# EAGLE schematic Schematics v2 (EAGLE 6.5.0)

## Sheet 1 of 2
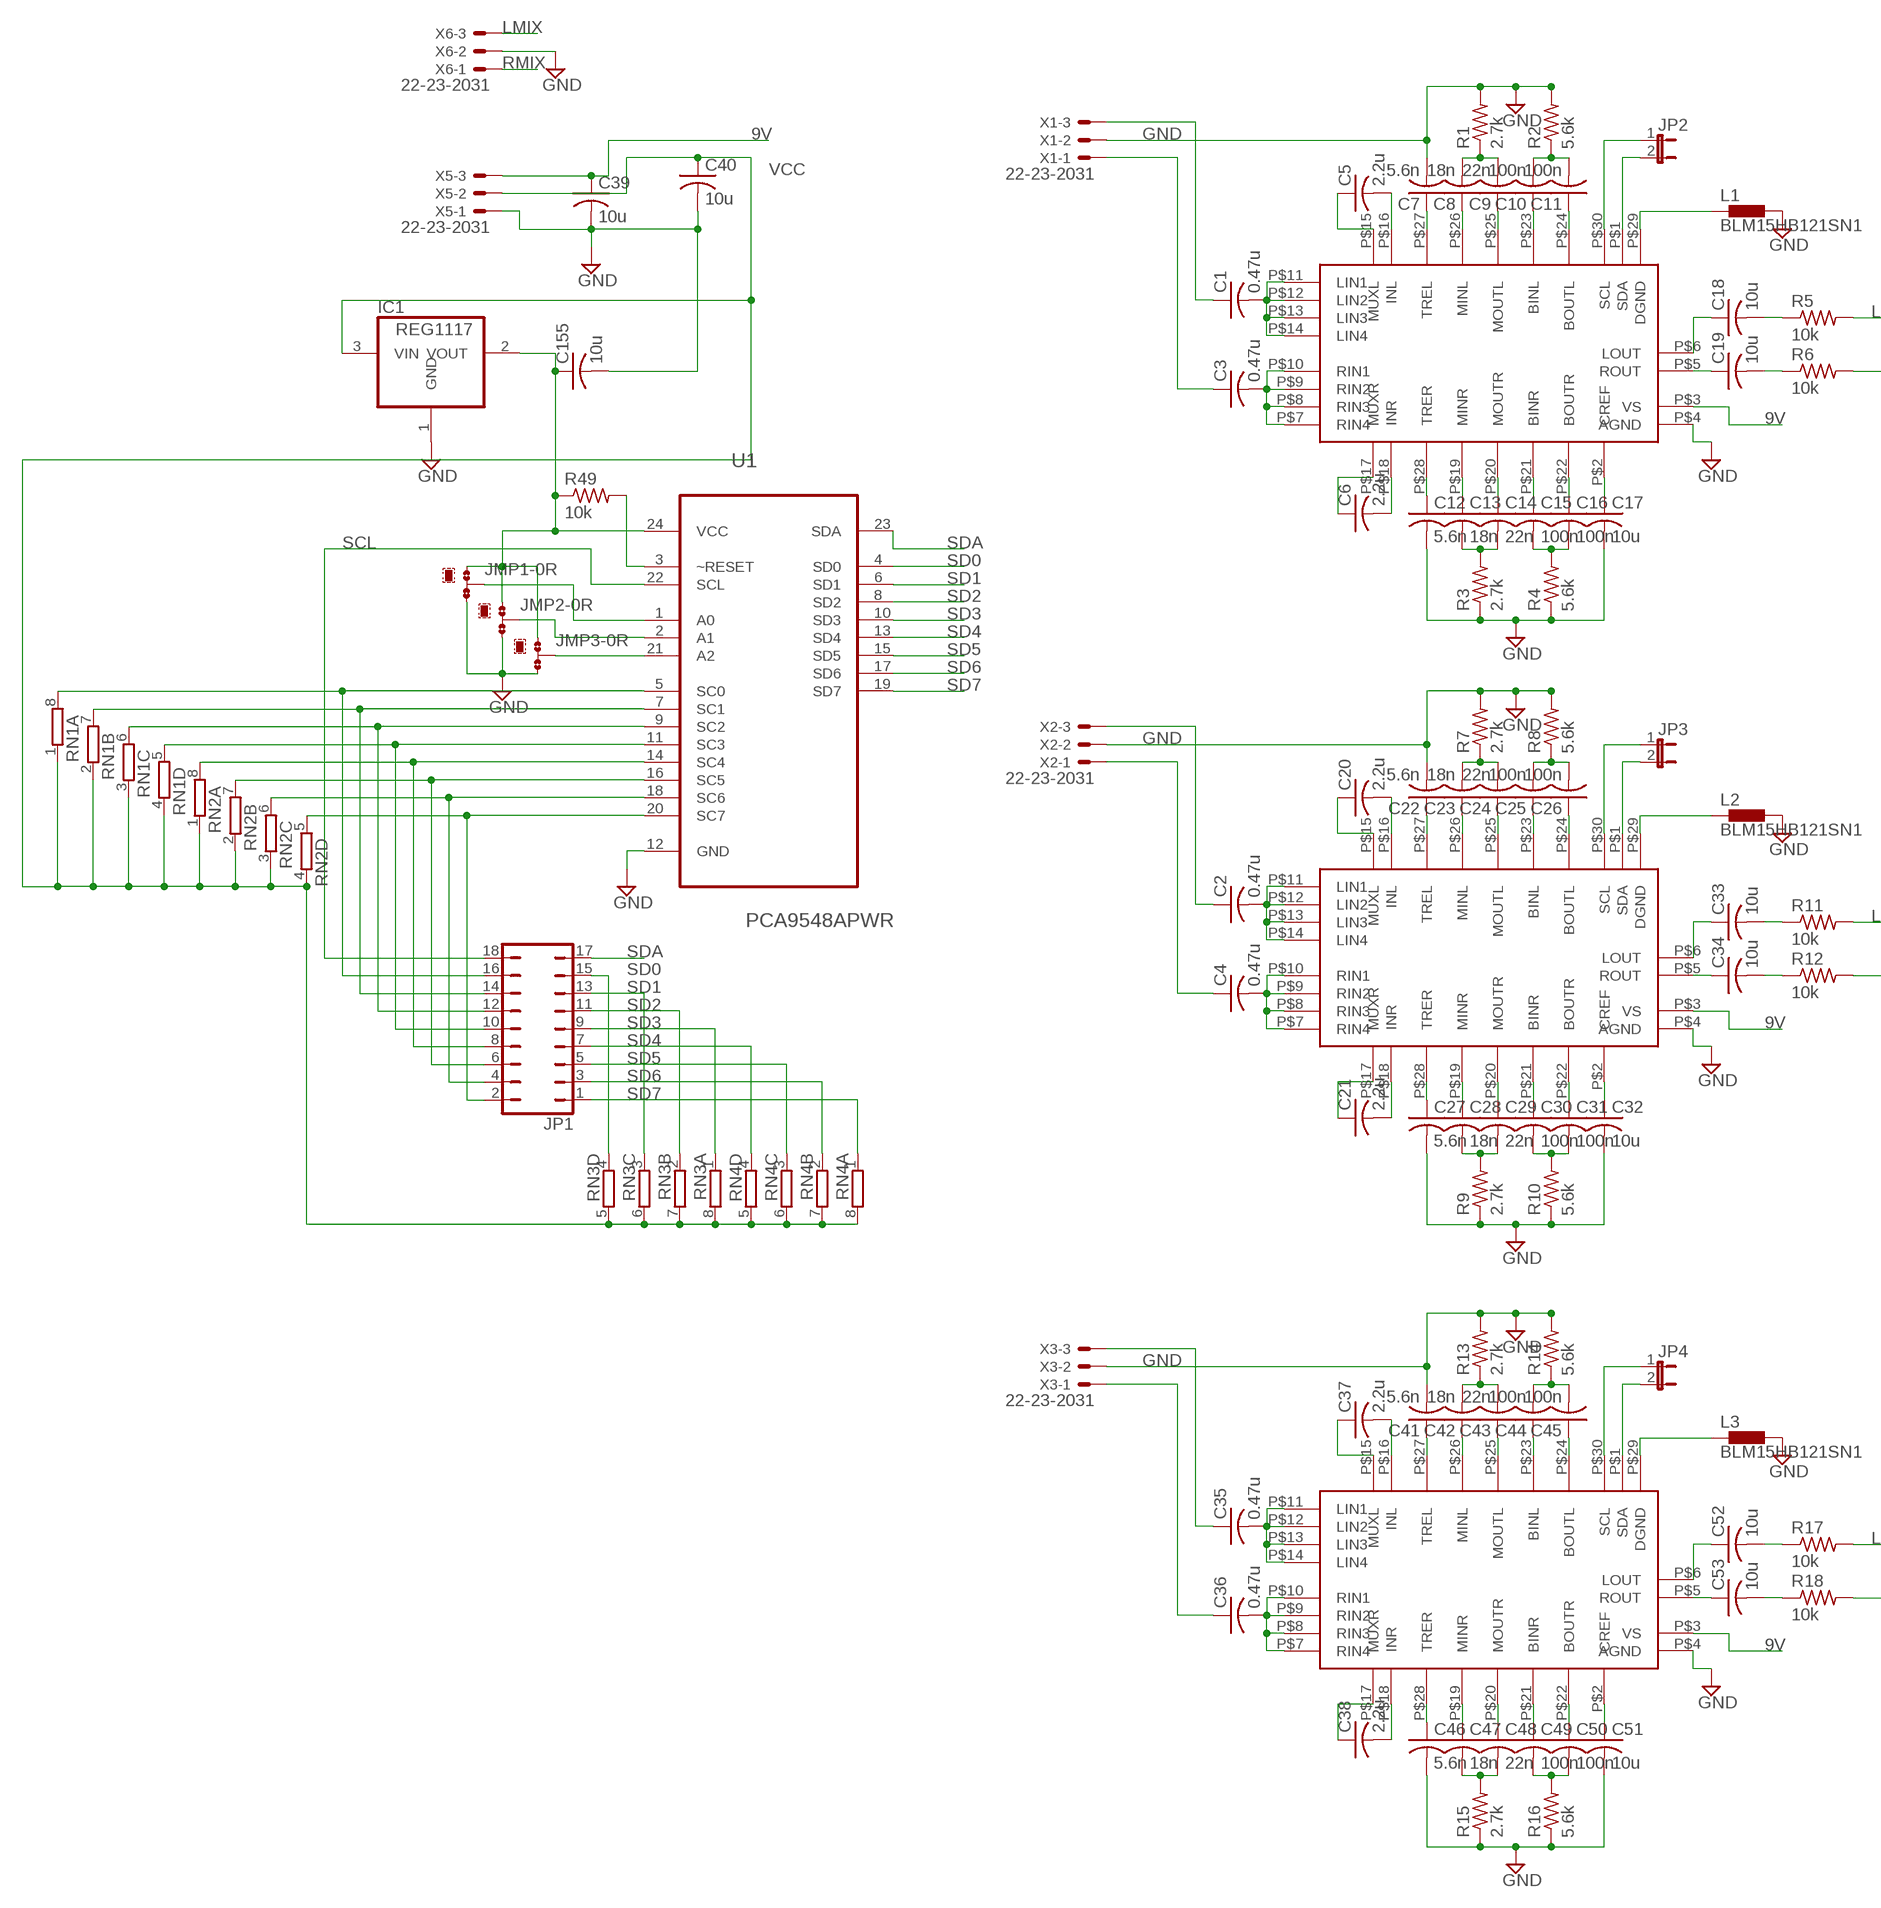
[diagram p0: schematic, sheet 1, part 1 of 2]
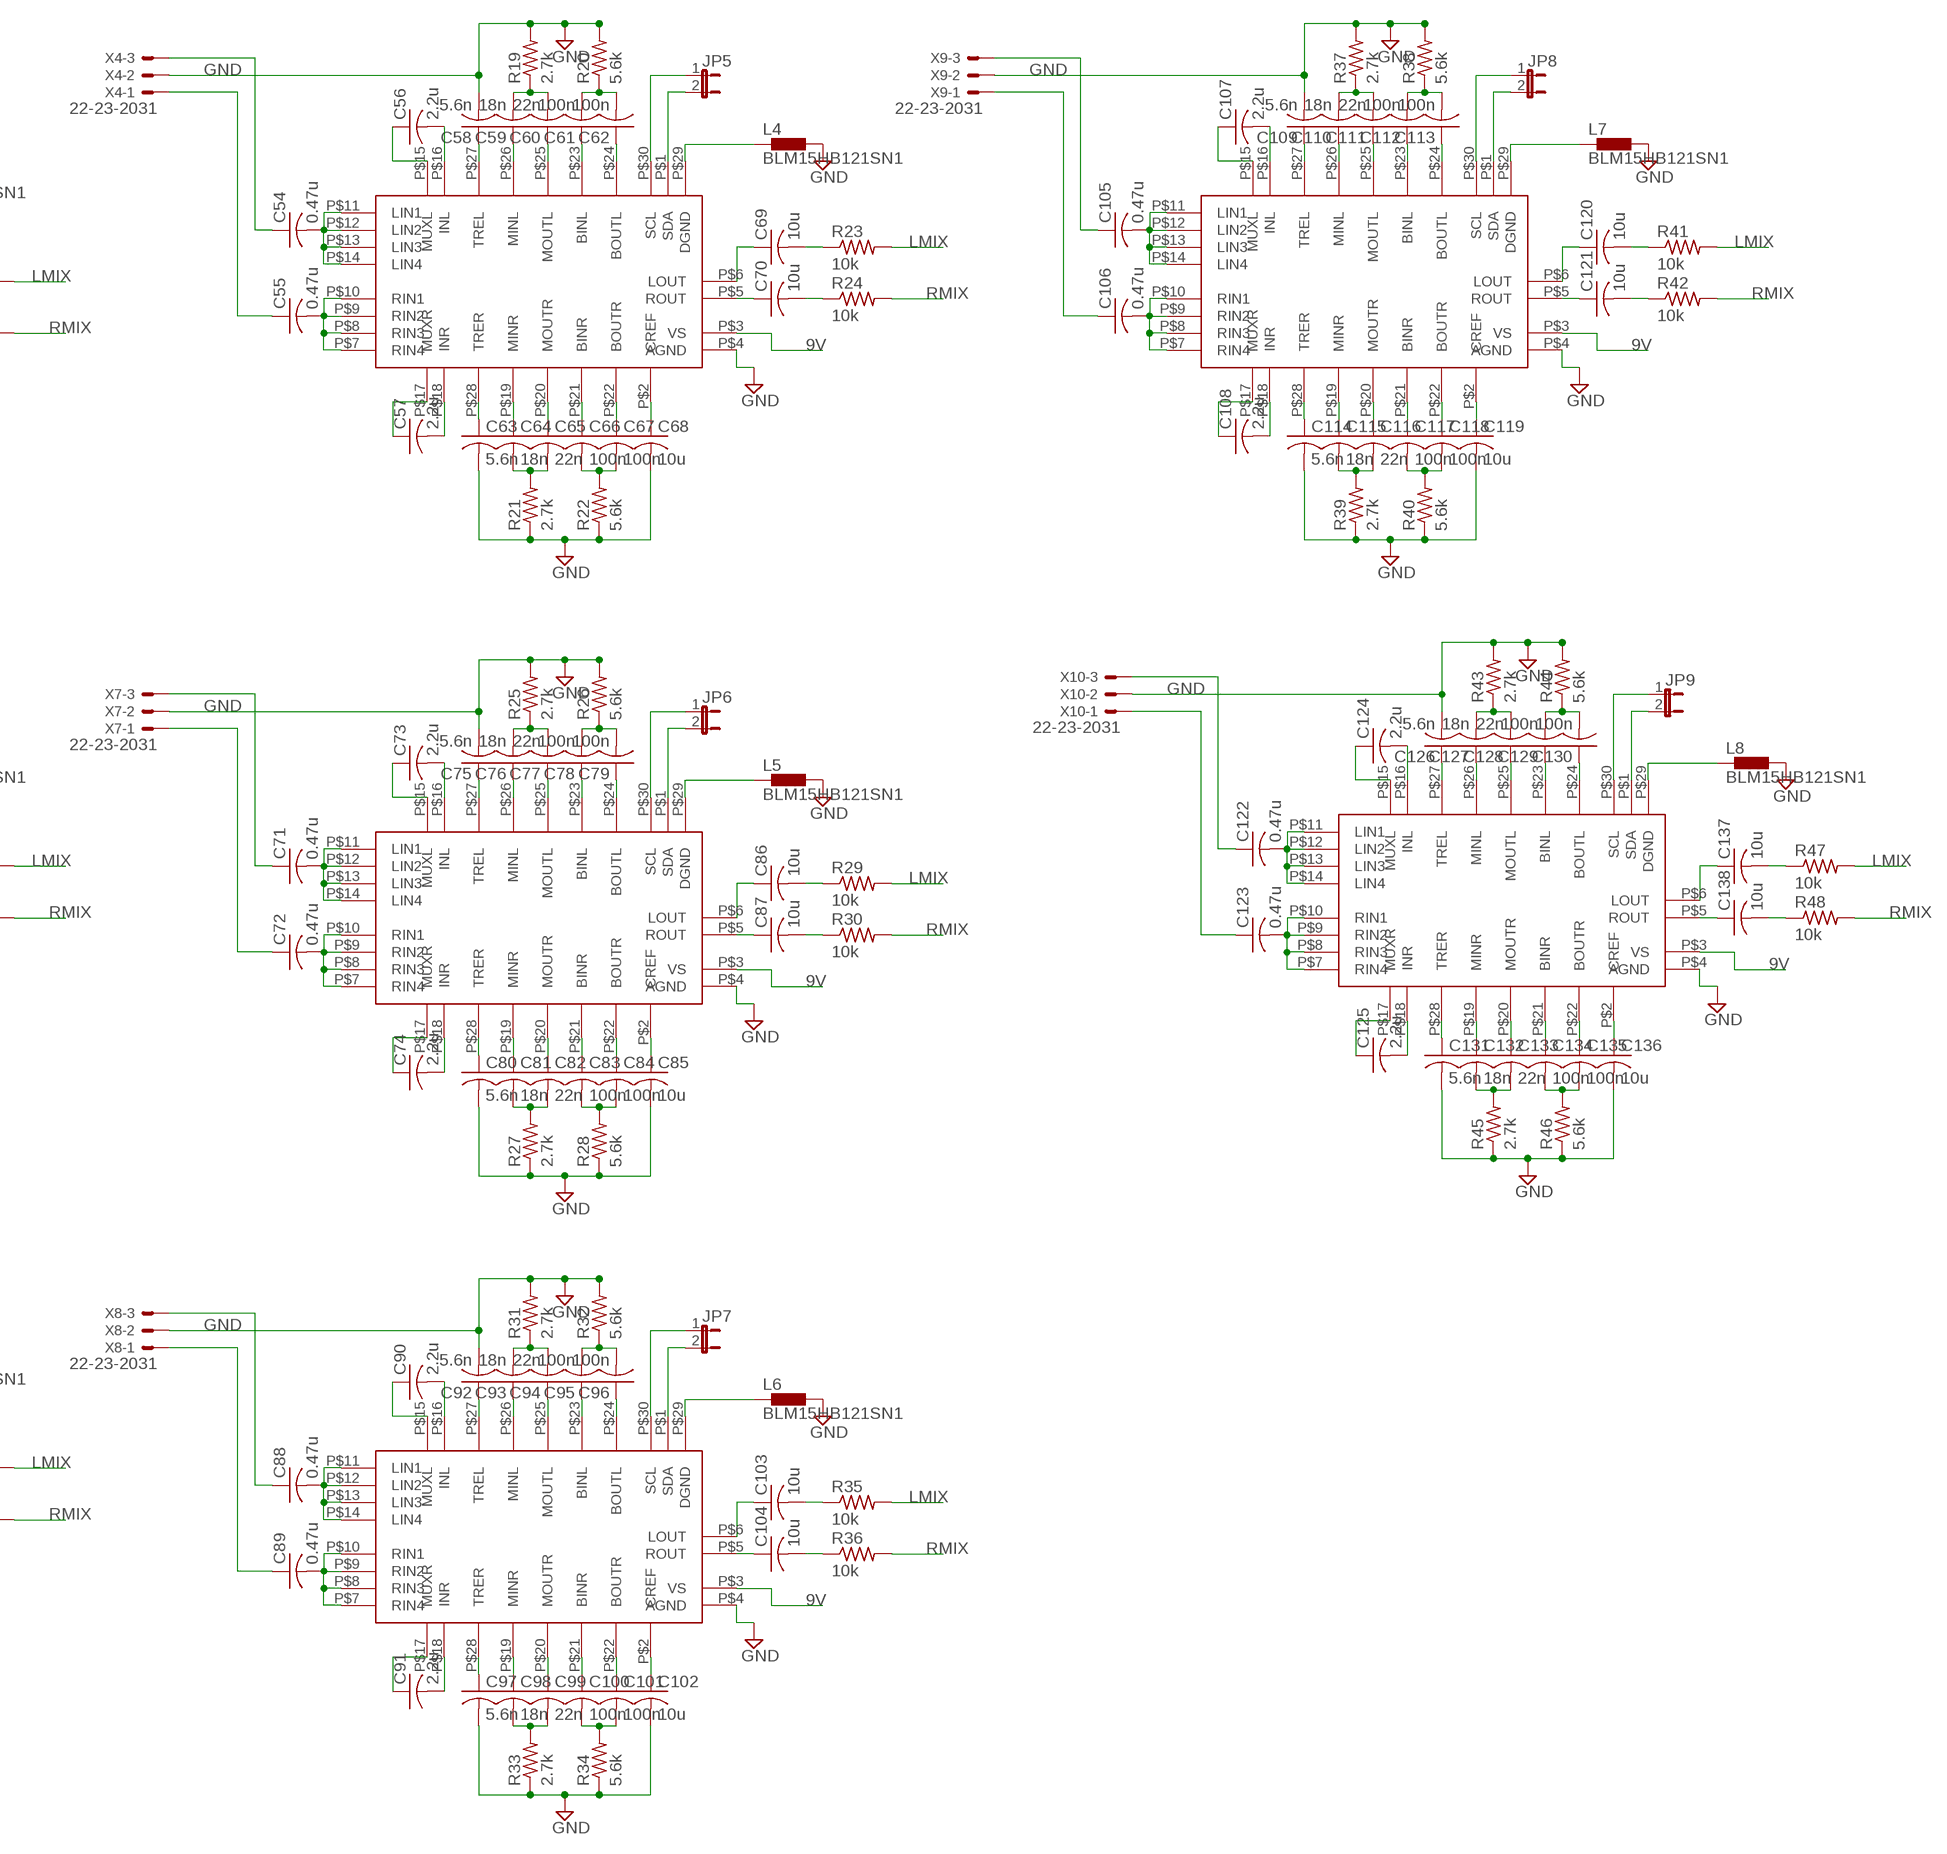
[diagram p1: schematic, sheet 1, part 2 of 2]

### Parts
C1  0.47u  C-USC0603K  [C0603K]
C2  0.47u  C-USC0603K  [C0603K]
C3  0.47u  C-USC0603K  [C0603K]
C4  0.47u  C-USC0603K  [C0603K]
C5  2.2u  C-USC0603K  [C0603K]
C6  2.2u  C-USC0603K  [C0603K]
C7  5.6n  C-USC0603K  [C0603K]
C8  18n  C-USC0603K  [C0603K]
C9  22n  C-USC0603K  [C0603K]
C10  100n  C-USC0603K  [C0603K]
C11  100n  C-USC0603K  [C0603K]
C12  5.6n  C-USC0603K  [C0603K]
C13  18n  C-USC0603K  [C0603K]
C14  22n  C-USC0603K  [C0603K]
C15  100n  C-USC0603K  [C0603K]
C16  100n  C-USC0603K  [C0603K]
C17  10u  C-USC0603K  [C0603K]
C18  10u  C-USC1206  [C1206]
C19  10u  C-USC1206  [C1206]
C20  2.2u  C-USC0603K  [C0603K]
C21  2.2u  C-USC0603K  [C0603K]
C22  5.6n  C-USC0603K  [C0603K]
C23  18n  C-USC0603K  [C0603K]
C24  22n  C-USC0603K  [C0603K]
C25  100n  C-USC0603K  [C0603K]
C26  100n  C-USC0603K  [C0603K]
C27  5.6n  C-USC0603K  [C0603K]
C28  18n  C-USC0603K  [C0603K]
C29  22n  C-USC0603K  [C0603K]
C30  100n  C-USC0603K  [C0603K]
C31  100n  C-USC0603K  [C0603K]
C32  10u  C-USC0603K  [C0603K]
C33  10u  C-USC1206  [C1206]
C34  10u  C-USC1206  [C1206]
C35  0.47u  C-USC0603K  [C0603K]
C36  0.47u  C-USC0603K  [C0603K]
C37  2.2u  C-USC0603K  [C0603K]
C38  2.2u  C-USC0603K  [C0603K]
C39  10u  C-USC1206  [C1206]
C40  10u  C-USC1206  [C1206]
C41  5.6n  C-USC0603K  [C0603K]
C42  18n  C-USC0603K  [C0603K]
C43  22n  C-USC0603K  [C0603K]
C44  100n  C-USC0603K  [C0603K]
C45  100n  C-USC0603K  [C0603K]
C46  5.6n  C-USC0603K  [C0603K]
C47  18n  C-USC0603K  [C0603K]
C48  22n  C-USC0603K  [C0603K]
C49  100n  C-USC0603K  [C0603K]
C50  100n  C-USC0603K  [C0603K]
C51  10u  C-USC0603K  [C0603K]
C52  10u  C-USC1206  [C1206]
C53  10u  C-USC1206  [C1206]
C54  0.47u  C-USC0603K  [C0603K]
C55  0.47u  C-USC0603K  [C0603K]
C56  2.2u  C-USC0603K  [C0603K]
C57  2.2u  C-USC0603K  [C0603K]
C58  5.6n  C-USC0603K  [C0603K]
C59  18n  C-USC0603K  [C0603K]
C60  22n  C-USC0603K  [C0603K]
C61  100n  C-USC0603K  [C0603K]
C62  100n  C-USC0603K  [C0603K]
C63  5.6n  C-USC0603K  [C0603K]
C64  18n  C-USC0603K  [C0603K]
C65  22n  C-USC0603K  [C0603K]
C66  100n  C-USC0603K  [C0603K]
C67  100n  C-USC0603K  [C0603K]
C68  10u  C-USC0603K  [C0603K]
C69  10u  C-USC1206  [C1206]
C70  10u  C-USC1206  [C1206]
C71  0.47u  C-USC0603K  [C0603K]
C72  0.47u  C-USC0603K  [C0603K]
C73  2.2u  C-USC0603K  [C0603K]
C74  2.2u  C-USC0603K  [C0603K]
C75  5.6n  C-USC0603K  [C0603K]
C76  18n  C-USC0603K  [C0603K]
C77  22n  C-USC0603K  [C0603K]
C78  100n  C-USC0603K  [C0603K]
C79  100n  C-USC0603K  [C0603K]
C80  5.6n  C-USC0603K  [C0603K]
C81  18n  C-USC0603K  [C0603K]
C82  22n  C-USC0603K  [C0603K]
C83  100n  C-USC0603K  [C0603K]
C84  100n  C-USC0603K  [C0603K]
C85  10u  C-USC0603K  [C0603K]
C86  10u  C-USC1206  [C1206]
C87  10u  C-USC1206  [C1206]
C88  0.47u  C-USC0603K  [C0603K]
C89  0.47u  C-USC0603K  [C0603K]
C90  2.2u  C-USC0603K  [C0603K]
C91  2.2u  C-USC0603K  [C0603K]
C92  5.6n  C-USC0603K  [C0603K]
C93  18n  C-USC0603K  [C0603K]
C94  22n  C-USC0603K  [C0603K]
C95  100n  C-USC0603K  [C0603K]
C96  100n  C-USC0603K  [C0603K]
C97  5.6n  C-USC0603K  [C0603K]
C98  18n  C-USC0603K  [C0603K]
C99  22n  C-USC0603K  [C0603K]
C100  100n  C-USC0603K  [C0603K]
C101  100n  C-USC0603K  [C0603K]
C102  10u  C-USC0603K  [C0603K]
C103  10u  C-USC1206  [C1206]
C104  10u  C-USC1206  [C1206]
C105  0.47u  C-USC0603K  [C0603K]
C106  0.47u  C-USC0603K  [C0603K]
C107  2.2u  C-USC0603K  [C0603K]
C108  2.2u  C-USC0603K  [C0603K]
C109  5.6n  C-USC0603K  [C0603K]
C110  18n  C-USC0603K  [C0603K]
C111  22n  C-USC0603K  [C0603K]
C112  100n  C-USC0603K  [C0603K]
C113  100n  C-USC0603K  [C0603K]
C114  5.6n  C-USC0603K  [C0603K]
C115  18n  C-USC0603K  [C0603K]
C116  22n  C-USC0603K  [C0603K]
C117  100n  C-USC0603K  [C0603K]
C118  100n  C-USC0603K  [C0603K]
C119  10u  C-USC0603K  [C0603K]
C120  10u  C-USC1206  [C1206]
C121  10u  C-USC1206  [C1206]
C122  0.47u  C-USC0603K  [C0603K]
C123  0.47u  C-USC0603K  [C0603K]
C124  2.2u  C-USC0603K  [C0603K]
C125  2.2u  C-USC0603K  [C0603K]
C126  5.6n  C-USC0603K  [C0603K]
C127  18n  C-USC0603K  [C0603K]
C128  22n  C-USC0603K  [C0603K]
C129  100n  C-USC0603K  [C0603K]
C130  100n  C-USC0603K  [C0603K]
C131  5.6n  C-USC0603K  [C0603K]
C132  18n  C-USC0603K  [C0603K]
C133  22n  C-USC0603K  [C0603K]
C134  100n  C-USC0603K  [C0603K]
C135  100n  C-USC0603K  [C0603K]
C136  10u  C-USC0603K  [C0603K]
C137  10u  C-USC1206  [C1206]
C138  10u  C-USC1206  [C1206]
C155  10u  C-USC1206  [C1206]
IC1  REG1117  [SOT223]
JMP1  0R-JUMPB  [B0R-JMP]
JMP2  0R-JUMPB  [B0R-JMP]
JMP3  0R-JUMPB  [B0R-JMP]
JP1  JP9Q  [JP9Q]
JP2  JP1E  [JP1]
JP3  JP1E  [JP1]
JP4  JP1E  [JP1]
JP5  JP1E  [JP1]
JP6  JP1E  [JP1]
JP7  JP1E  [JP1]
JP8  JP1E  [JP1]
JP9  JP1E  [JP1]
L1  BLM15HB121SN1  [0402]
L2  BLM15HB121SN1  [0402]
L3  BLM15HB121SN1  [0402]
L4  BLM15HB121SN1  [0402]
L5  BLM15HB121SN1  [0402]
L6  BLM15HB121SN1  [0402]
L7  BLM15HB121SN1  [0402]
L8  BLM15HB121SN1  [0402]
R1  2.7k  R-US_M0805  [M0805]
R2  5.6k  R-US_M0805  [M0805]
R3  2.7k  R-US_M0805  [M0805]
R4  5.6k  R-US_M0805  [M0805]
R5  10k  R-US_R1206  [R1206]
R6  10k  R-US_R1206  [R1206]
R7  2.7k  R-US_M0805  [M0805]
R8  5.6k  R-US_M0805  [M0805]
R9  2.7k  R-US_M0805  [M0805]
R10  5.6k  R-US_M0805  [M0805]
R11  10k  R-US_R1206  [R1206]
R12  10k  R-US_R1206  [R1206]
R13  2.7k  R-US_M0805  [M0805]
R14  5.6k  R-US_M0805  [M0805]
R15  2.7k  R-US_M0805  [M0805]
R16  5.6k  R-US_M0805  [M0805]
R17  10k  R-US_R1206  [R1206]
R18  10k  R-US_R1206  [R1206]
R19  2.7k  R-US_M0805  [M0805]
R20  5.6k  R-US_M0805  [M0805]
R21  2.7k  R-US_M0805  [M0805]
R22  5.6k  R-US_M0805  [M0805]
R23  10k  R-US_R1206  [R1206]
R24  10k  R-US_R1206  [R1206]
R25  2.7k  R-US_M0805  [M0805]
R26  5.6k  R-US_M0805  [M0805]
R27  2.7k  R-US_M0805  [M0805]
R28  5.6k  R-US_M0805  [M0805]
R29  10k  R-US_R1206  [R1206]
R30  10k  R-US_R1206  [R1206]
R31  2.7k  R-US_M0805  [M0805]
R32  5.6k  R-US_M0805  [M0805]
R33  2.7k  R-US_M0805  [M0805]
R34  5.6k  R-US_M0805  [M0805]
R35  10k  R-US_R1206  [R1206]
R36  10k  R-US_R1206  [R1206]
R37  2.7k  R-US_M0805  [M0805]
R38  5.6k  R-US_M0805  [M0805]
R39  2.7k  R-US_M0805  [M0805]
R40  5.6k  R-US_M0805  [M0805]
R41  10k  R-US_R1206  [R1206]
R42  10k  R-US_R1206  [R1206]
R43  2.7k  R-US_M0805  [M0805]
R44  5.6k  R-US_M0805  [M0805]
R45  2.7k  R-US_M0805  [M0805]
R46  5.6k  R-US_M0805  [M0805]
R47  10k  R-US_R1206  [R1206]
R48  10k  R-US_R1206  [R1206]
R49  10k  R-US_R1206  [R1206]
RN1  4R-NCAY16  [CAY16]
RN2  4R-NCAY16  [CAY16]
RN3  4R-NCAY16  [CAY16]
RN4  4R-NCAY16  [CAY16]
U1  PCA9548APWR  [SOP65P640X120-24N]
U$1  TDA7439  [SDIP30]
U$2  TDA7439  [SDIP30]
U$3  TDA7439  [SDIP30]
U$4  TDA7439  [SDIP30]
U$5  TDA7439  [SDIP30]
U$6  TDA7439  [SDIP30]
U$7  TDA7439  [SDIP30]
U$8  TDA7439  [SDIP30]
X1  22-23-2031  [22-23-2031]
X2  22-23-2031  [22-23-2031]
X3  22-23-2031  [22-23-2031]
X4  22-23-2031  [22-23-2031]
X5  22-23-2031  [22-23-2031]
X6  22-23-2031  [22-23-2031]
X7  22-23-2031  [22-23-2031]
X8  22-23-2031  [22-23-2031]
X9  22-23-2031  [22-23-2031]
X10  22-23-2031  [22-23-2031]

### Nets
3.3V: C155.1 IC1.2(VOUT) JMP1.1 JMP2.1 JMP3.1 R49.1 U1.24(VCC)
9V: C39.1 U$1.P$3(VS) U$2.P$3(VS) U$3.P$3(VS) U$4.P$3(VS) U$5.P$3(VS) U$6.P$3(VS) U$7.P$3(VS) U$8.P$3(VS) X5.3 ; also sheet 2
GND: C7.2 C12.2 C17.2 C22.2 C27.2 C32.2 C39.2 C40.2 C41.2 C46.2 C51.2 C58.2 C63.2 C68.2 C75.2 C80.2 C85.2 C92.2 C97.2 C102.2 C109.2 C114.2 C119.2 C126.2 C131.2 C136.2 C155.2 IC1.1(GND) JMP1.3 JMP2.3 JMP3.3 L1.2 L2.2 L3.2 L4.2 L5.2 L6.2 L7.2 L8.2 R1.2 R2.2 R3.1 R4.1 R7.2 R8.2 R9.1 R10.1 R13.2 R14.2 R15.1 R16.1 R19.2 R20.2 R21.1 R22.1 R25.2 R26.2 R27.1 R28.1 R31.2 R32.2 R33.1 R34.1 R37.2 R38.2 R39.1 R40.1 R43.2 R44.2 R45.1 R46.1 U1.12(GND) U$1.P$4(AGND) U$2.P$4(AGND) U$3.P$4(AGND) U$4.P$4(AGND) U$5.P$4(AGND) U$6.P$4(AGND) U$7.P$4(AGND) U$8.P$4(AGND) X1.2 X2.2 X3.2 X4.2 X5.1 X6.2 X7.2 X8.2 X9.2 X10.2 ; also sheet 2
LMIX: R5.2 R11.2 R17.2 R23.2 R29.2 R35.2 R41.2 R47.2 X6.3 ; also sheet 2
N$1: C1.1 X1.3
N$2: C1.2 U$1.P$11(LIN1) U$1.P$12(LIN2) U$1.P$13(LIN3) U$1.P$14(LIN4)
N$3: C3.1 X1.1
N$4: C3.2 U$1.P$7(RIN4) U$1.P$8(RIN3) U$1.P$9(RIN2) U$1.P$10(RIN1)
N$5: C5.1 U$1.P$15(MUXL)
N$6: C5.2 U$1.P$16(INL)
N$7: C6.1 U$1.P$17(MUXR)
N$8: C6.2 U$1.P$18(INR)
N$9: C7.1 U$1.P$27(TREL)
N$10: C8.1 U$1.P$26(MINL)
N$11: C9.1 U$1.P$25(MOUTL)
N$12: C10.1 U$1.P$23(BINL)
N$13: C11.1 U$1.P$24(BOUTL)
N$14: C12.1 U$1.P$28(TRER)
N$15: C13.1 U$1.P$19(MINR)
N$16: C14.1 U$1.P$20(MOUTR)
N$17: C15.1 U$1.P$21(BINR)
N$18: C16.1 U$1.P$22(BOUTR)
N$19: C17.1 U$1.P$2(CREF)
N$20: C8.2 C9.2 R1.1
N$21: C10.2 C11.2 R2.1
N$22: C13.2 C14.2 R3.2
N$23: C15.2 C16.2 R4.2
N$24: JP2.1 U$1.P$30(SCL)
N$25: JP2.2 U$1.P$1(SDA)
N$26: L1.1 U$1.P$29(DGND)
N$27: C18.1 U$1.P$6(LOUT)
N$28: C19.1 U$1.P$5(ROUT)
N$29: C18.2 R5.1
N$30: C19.2 R6.1
N$31: C2.2 U$2.P$11(LIN1) U$2.P$12(LIN2) U$2.P$13(LIN3) U$2.P$14(LIN4)
N$32: C4.2 U$2.P$7(RIN4) U$2.P$8(RIN3) U$2.P$9(RIN2) U$2.P$10(RIN1)
N$33: C20.1 U$2.P$15(MUXL)
N$34: C20.2 U$2.P$16(INL)
N$35: C21.1 U$2.P$17(MUXR)
N$36: C21.2 U$2.P$18(INR)
N$37: C22.1 U$2.P$27(TREL)
N$38: C23.1 U$2.P$26(MINL)
N$39: C24.1 U$2.P$25(MOUTL)
N$40: C25.1 U$2.P$23(BINL)
N$41: C26.1 U$2.P$24(BOUTL)
N$42: C27.1 U$2.P$28(TRER)
N$43: C28.1 U$2.P$19(MINR)
N$44: C29.1 U$2.P$20(MOUTR)
N$45: C30.1 U$2.P$21(BINR)
N$46: C31.1 U$2.P$22(BOUTR)
N$47: C32.1 U$2.P$2(CREF)
N$48: C23.2 C24.2 R7.1
N$49: C25.2 C26.2 R8.1
N$50: C28.2 C29.2 R9.2
N$51: C30.2 C31.2 R10.2
N$52: C33.1 U$2.P$6(LOUT)
N$53: C34.1 U$2.P$5(ROUT)
N$54: C33.2 R11.1
N$55: C34.2 R12.1
N$56: C4.1 X2.1
N$57: JP3.1 U$2.P$30(SCL)
N$58: JP3.2 U$2.P$1(SDA)
N$59: C2.1 X2.3
N$60: L2.1 U$2.P$29(DGND)
N$61: C35.2 U$3.P$11(LIN1) U$3.P$12(LIN2) U$3.P$13(LIN3) U$3.P$14(LIN4)
N$62: C36.2 U$3.P$7(RIN4) U$3.P$8(RIN3) U$3.P$9(RIN2) U$3.P$10(RIN1)
N$63: C37.1 U$3.P$15(MUXL)
N$64: C37.2 U$3.P$16(INL)
N$65: C38.1 U$3.P$17(MUXR)
N$66: C38.2 U$3.P$18(INR)
N$67: C41.1 U$3.P$27(TREL)
N$68: C42.1 U$3.P$26(MINL)
N$69: C43.1 U$3.P$25(MOUTL)
N$70: C44.1 U$3.P$23(BINL)
N$71: C45.1 U$3.P$24(BOUTL)
N$72: C46.1 U$3.P$28(TRER)
N$73: C47.1 U$3.P$19(MINR)
N$74: C48.1 U$3.P$20(MOUTR)
N$75: C49.1 U$3.P$21(BINR)
N$76: C50.1 U$3.P$22(BOUTR)
N$77: C51.1 U$3.P$2(CREF)
N$78: C42.2 C43.2 R13.1
N$79: C44.2 C45.2 R14.1
N$80: C47.2 C48.2 R15.2
N$81: C49.2 C50.2 R16.2
N$82: C52.1 U$3.P$6(LOUT)
N$83: C53.1 U$3.P$5(ROUT)
N$84: C52.2 R17.1
N$85: C53.2 R18.1
N$86: C36.1 X3.1
N$87: JP4.1 U$3.P$30(SCL)
N$88: JP4.2 U$3.P$1(SDA)
N$89: C35.1 X3.3
N$90: L3.1 U$3.P$29(DGND)
N$91: C54.2 U$4.P$11(LIN1) U$4.P$12(LIN2) U$4.P$13(LIN3) U$4.P$14(LIN4)
N$92: C55.2 U$4.P$7(RIN4) U$4.P$8(RIN3) U$4.P$9(RIN2) U$4.P$10(RIN1)
N$93: C56.1 U$4.P$15(MUXL)
N$94: C56.2 U$4.P$16(INL)
N$95: C57.1 U$4.P$17(MUXR)
N$96: C57.2 U$4.P$18(INR)
N$97: C58.1 U$4.P$27(TREL)
N$98: C59.1 U$4.P$26(MINL)
N$99: C60.1 U$4.P$25(MOUTL)
N$100: C61.1 U$4.P$23(BINL)
N$101: C62.1 U$4.P$24(BOUTL)
N$102: C63.1 U$4.P$28(TRER)
N$103: C64.1 U$4.P$19(MINR)
N$104: C65.1 U$4.P$20(MOUTR)
N$105: C66.1 U$4.P$21(BINR)
N$106: C67.1 U$4.P$22(BOUTR)
N$107: C68.1 U$4.P$2(CREF)
N$108: C59.2 C60.2 R19.1
N$109: C61.2 C62.2 R20.1
N$110: C64.2 C65.2 R21.2
N$111: C66.2 C67.2 R22.2
N$112: C69.1 U$4.P$6(LOUT)
N$113: C70.1 U$4.P$5(ROUT)
N$114: C69.2 R23.1
N$115: C70.2 R24.1
N$116: C55.1 X4.1
N$117: JP5.1 U$4.P$30(SCL)
N$118: JP5.2 U$4.P$1(SDA)
N$119: C54.1 X4.3
N$120: L4.1 U$4.P$29(DGND)
N$121: C71.2 U$5.P$11(LIN1) U$5.P$12(LIN2) U$5.P$13(LIN3) U$5.P$14(LIN4)
N$122: C72.2 U$5.P$7(RIN4) U$5.P$8(RIN3) U$5.P$9(RIN2) U$5.P$10(RIN1)
N$123: C73.1 U$5.P$15(MUXL)
N$124: C73.2 U$5.P$16(INL)
N$125: C74.1 U$5.P$17(MUXR)
N$126: C74.2 U$5.P$18(INR)
N$127: C75.1 U$5.P$27(TREL)
N$128: C76.1 U$5.P$26(MINL)
N$129: C77.1 U$5.P$25(MOUTL)
N$130: C78.1 U$5.P$23(BINL)
N$131: C79.1 U$5.P$24(BOUTL)
N$132: C80.1 U$5.P$28(TRER)
N$133: C81.1 U$5.P$19(MINR)
N$134: C82.1 U$5.P$20(MOUTR)
N$135: C83.1 U$5.P$21(BINR)
N$136: C84.1 U$5.P$22(BOUTR)
N$137: C85.1 U$5.P$2(CREF)
N$138: C76.2 C77.2 R25.1
N$139: C78.2 C79.2 R26.1
N$140: C81.2 C82.2 R27.2
N$141: C83.2 C84.2 R28.2
N$142: C86.1 U$5.P$6(LOUT)
N$143: C87.1 U$5.P$5(ROUT)
N$144: C86.2 R29.1
N$145: C87.2 R30.1
N$146: C72.1 X7.1
N$147: JP6.1 U$5.P$30(SCL)
N$148: JP6.2 U$5.P$1(SDA)
N$149: C71.1 X7.3
N$150: L5.1 U$5.P$29(DGND)
N$151: C88.2 U$6.P$11(LIN1) U$6.P$12(LIN2) U$6.P$13(LIN3) U$6.P$14(LIN4)
N$152: C89.2 U$6.P$7(RIN4) U$6.P$8(RIN3) U$6.P$9(RIN2) U$6.P$10(RIN1)
N$153: C90.1 U$6.P$15(MUXL)
N$154: C90.2 U$6.P$16(INL)
N$155: C91.1 U$6.P$17(MUXR)
N$156: C91.2 U$6.P$18(INR)
N$157: C92.1 U$6.P$27(TREL)
N$158: C93.1 U$6.P$26(MINL)
N$159: C94.1 U$6.P$25(MOUTL)
N$160: C95.1 U$6.P$23(BINL)
N$161: C96.1 U$6.P$24(BOUTL)
N$162: C97.1 U$6.P$28(TRER)
N$163: C98.1 U$6.P$19(MINR)
N$164: C99.1 U$6.P$20(MOUTR)
N$165: C100.1 U$6.P$21(BINR)
N$166: C101.1 U$6.P$22(BOUTR)
N$167: C102.1 U$6.P$2(CREF)
N$168: C93.2 C94.2 R31.1
N$169: C95.2 C96.2 R32.1
N$170: C98.2 C99.2 R33.2
N$171: C100.2 C101.2 R34.2
N$172: C103.1 U$6.P$6(LOUT)
N$173: C104.1 U$6.P$5(ROUT)
N$174: C103.2 R35.1
N$175: C104.2 R36.1
N$176: C89.1 X8.1
N$177: JP7.1 U$6.P$30(SCL)
N$178: JP7.2 U$6.P$1(SDA)
N$179: C88.1 X8.3
N$180: L6.1 U$6.P$29(DGND)
N$181: C105.2 U$7.P$11(LIN1) U$7.P$12(LIN2) U$7.P$13(LIN3) U$7.P$14(LIN4)
N$182: C106.2 U$7.P$7(RIN4) U$7.P$8(RIN3) U$7.P$9(RIN2) U$7.P$10(RIN1)
N$183: C107.1 U$7.P$15(MUXL)
N$184: C107.2 U$7.P$16(INL)
N$185: C108.1 U$7.P$17(MUXR)
N$186: C108.2 U$7.P$18(INR)
N$187: C109.1 U$7.P$27(TREL)
N$188: C110.1 U$7.P$26(MINL)
N$189: C111.1 U$7.P$25(MOUTL)
N$190: C112.1 U$7.P$23(BINL)
N$191: C113.1 U$7.P$24(BOUTL)
N$192: C114.1 U$7.P$28(TRER)
N$193: C115.1 U$7.P$19(MINR)
N$194: C116.1 U$7.P$20(MOUTR)
N$195: C117.1 U$7.P$21(BINR)
N$196: C118.1 U$7.P$22(BOUTR)
N$197: C119.1 U$7.P$2(CREF)
N$198: C110.2 C111.2 R37.1
N$199: C112.2 C113.2 R38.1
N$200: C115.2 C116.2 R39.2
N$201: C117.2 C118.2 R40.2
N$202: C120.1 U$7.P$6(LOUT)
N$203: C121.1 U$7.P$5(ROUT)
N$204: C120.2 R41.1
N$205: C121.2 R42.1
N$206: C106.1 X9.1
N$207: JP8.1 U$7.P$30(SCL)
N$208: JP8.2 U$7.P$1(SDA)
N$209: C105.1 X9.3
N$210: L7.1 U$7.P$29(DGND)
N$211: C122.2 U$8.P$11(LIN1) U$8.P$12(LIN2) U$8.P$13(LIN3) U$8.P$14(LIN4)
N$212: C123.2 U$8.P$7(RIN4) U$8.P$8(RIN3) U$8.P$9(RIN2) U$8.P$10(RIN1)
N$213: C124.1 U$8.P$15(MUXL)
N$214: C124.2 U$8.P$16(INL)
N$215: C125.1 U$8.P$17(MUXR)
N$216: C125.2 U$8.P$18(INR)
N$217: C126.1 U$8.P$27(TREL)
N$218: C127.1 U$8.P$26(MINL)
N$219: C128.1 U$8.P$25(MOUTL)
N$220: C129.1 U$8.P$23(BINL)
N$221: C130.1 U$8.P$24(BOUTL)
N$222: C131.1 U$8.P$28(TRER)
N$223: C132.1 U$8.P$19(MINR)
N$224: C133.1 U$8.P$20(MOUTR)
N$225: C134.1 U$8.P$21(BINR)
N$226: C135.1 U$8.P$22(BOUTR)
N$227: C136.1 U$8.P$2(CREF)
N$228: C127.2 C128.2 R43.1
N$229: C129.2 C130.2 R44.1
N$230: C132.2 C133.2 R45.2
N$231: C134.2 C135.2 R46.2
N$232: C137.1 U$8.P$6(LOUT)
N$233: C138.1 U$8.P$5(ROUT)
N$234: C137.2 R47.1
N$235: C138.2 R48.1
N$236: C123.1 X10.1
N$237: JP9.1 U$8.P$30(SCL)
N$238: JP9.2 U$8.P$1(SDA)
N$239: C122.1 X10.3
N$240: L8.1 U$8.P$29(DGND)
N$250: JP1.2 RN2.5 U1.20(SC7)
N$251: JP1.4 RN2.6 U1.18(SC6)
N$252: JP1.6 RN2.7 U1.16(SC5)
N$253: JP1.8 RN2.8 U1.14(SC4)
N$254: JP1.10 RN1.5 U1.11(SC3)
N$255: JP1.12 RN1.6 U1.9(SC2)
N$256: JP1.14 RN1.7 U1.7(SC1)
N$259: JP1.16 RN1.8 U1.5(SC0)
N$275: JMP1.2 U1.1(A0)
N$276: JMP2.2 U1.2(A1)
N$277: JMP3.2 U1.21(A2)
N$288: R49.2 U1.3(~RESET)
RMIX: R6.2 R12.2 R18.2 R24.2 R30.2 R36.2 R42.2 R48.2 X6.1 ; also sheet 2
SCL: JP1.18 U1.22(SCL)
SD0: JP1.15 RN3.4 U1.4(SD0)
SD1: JP1.13 RN3.3 U1.6(SD1)
SD2: JP1.11 RN3.2 U1.8(SD2)
SD3: JP1.9 RN3.1 U1.10(SD3)
SD4: JP1.7 RN4.4 U1.13(SD4)
SD5: JP1.5 RN4.3 U1.15(SD5)
SD6: JP1.3 RN4.2 U1.17(SD6)
SD7: JP1.1 RN4.1 U1.19(SD7)
SDA: JP1.17 U1.23(SDA)
VCC: C40.1 IC1.3(VIN) RN1.1 RN1.2 RN1.3 RN1.4 RN2.1 RN2.2 RN2.3 RN2.4 RN3.5 RN3.6 RN3.7 RN3.8 RN4.5 RN4.6 RN4.7 RN4.8 X5.2 ; also sheet 2

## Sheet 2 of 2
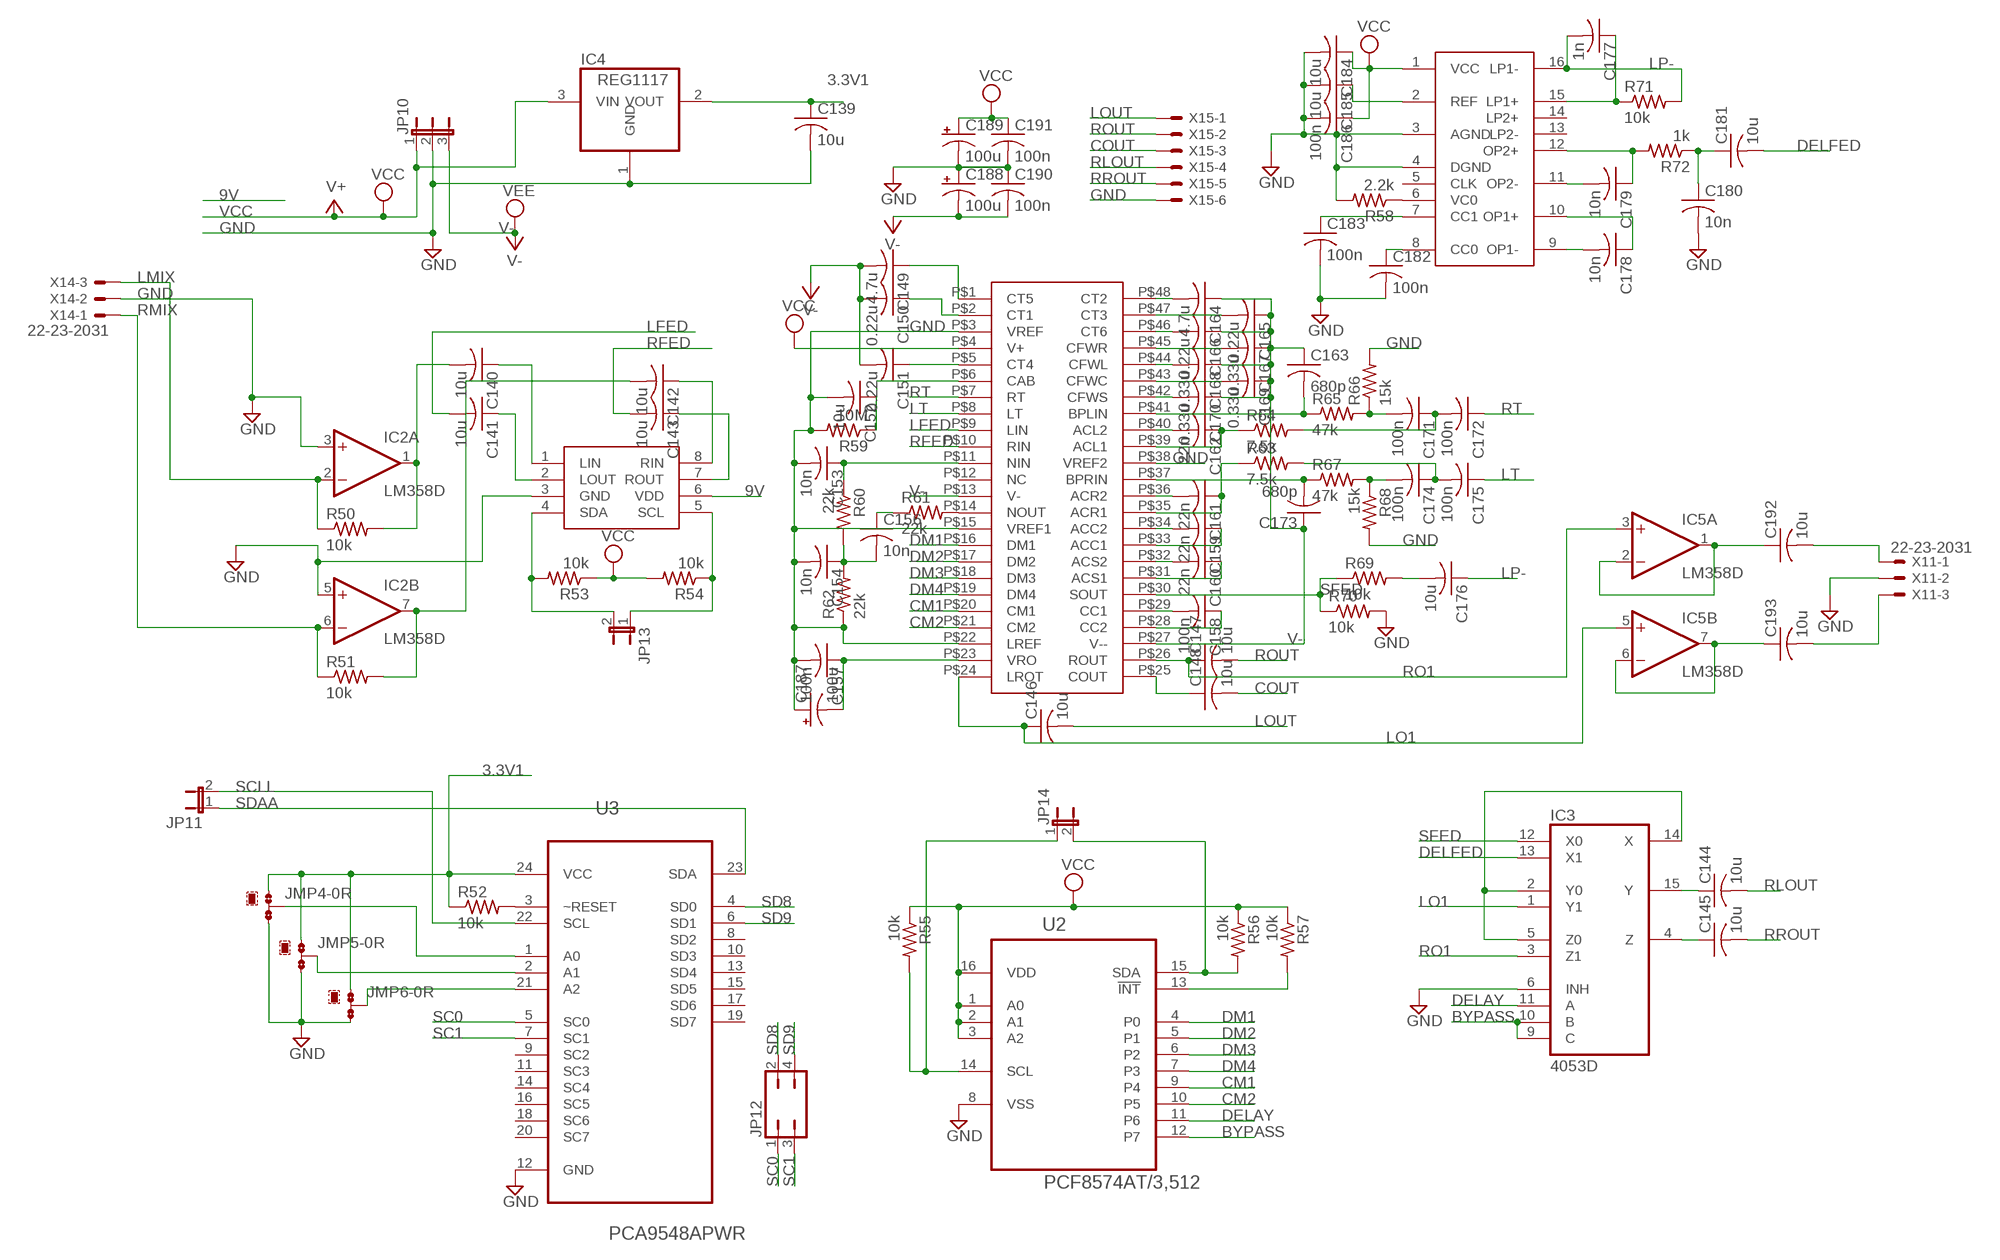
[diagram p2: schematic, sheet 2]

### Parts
C139  10u  C-USC1206  [C1206]
C140  10u  C-USC1206  [C1206]
C141  10u  C-USC1206  [C1206]
C142  10u  C-USC1206  [C1206]
C143  10u  C-USC1206  [C1206]
C144  10u  C-USC1206  [C1206]
C145  10u  C-USC1206  [C1206]
C146  10u  C-USC1206  [C1206]
C147  10u  C-USC1206  [C1206]
C148  10u  C-USC1206  [C1206]
C149  4.7u  C-USC1206  [C1206]
C150  0.22u  C-USC1206  [C1206]
C151  0.22u  C-USC1206  [C1206]
C152  10u  C-USC1206  [C1206]
C153  10n  C-USC1206  [C1206]
C154  10n  C-USC1206  [C1206]
C156  10n  C-USC1206  [C1206]
C157  100n  C-USC0603K  [C0603K]
C158  100n  C-USC0603K  [C0603K]
C159  22n  C-USC0603K  [C0603K]
C160  22n  C-USC0603K  [C0603K]
C161  22n  C-USC0603K  [C0603K]
C162  22n  C-USC0603K  [C0603K]
C163  680p  C-USC1206  [C1206]
C164  4.7u  C-USC1206  [C1206]
C165  0.22u  C-USC1206  [C1206]
C166  0.22u  C-USC1206  [C1206]
C167  0.33u  C-USC1206  [C1206]
C168  0.33u  C-USC1206  [C1206]
C169  0.33u  C-USC1206  [C1206]
C170  0.33u  C-USC1206  [C1206]
C171  100n  C-USC0603K  [C0603K]
C172  100n  C-USC0603K  [C0603K]
C173  680p  C-USC1206  [C1206]
C174  100n  C-USC0603K  [C0603K]
C175  100n  C-USC0603K  [C0603K]
C176  10u  C-USC1206  [C1206]
C177  1n  C-USC1206  [C1206]
C178  10n  C-USC1206  [C1206]
C179  10n  C-USC1206  [C1206]
C180  10n  C-USC1206  [C1206]
C181  10u  C-USC1206  [C1206]
C182  100n  C-USC0603K  [C0603K]
C183  100n  C-USC0603K  [C0603K]
C184  10u  C-USC1206  [C1206]
C185  10u  C-USC1206  [C1206]
C186  100n  C-USC0603K  [C0603K]
C187  100u  CPOL-USE2-5  [E2-5]
C188  100u  CPOL-USE2-5  [E2-5]
C189  100u  CPOL-USE2-5  [E2-5]
C190  100n  C-USC0603K  [C0603K]
C191  100n  C-USC0603K  [C0603K]
C192  10u  C-USC1206  [C1206]
C193  10u  C-USC1206  [C1206]
IC2  LM358D  [SO08]
IC3  4053D  [SO16]
IC4  REG1117  [SOT223]
IC5  LM358D  [SO08]
JMP4  0R-JUMPB  [B0R-JMP]
JMP5  0R-JUMPB  [B0R-JMP]
JMP6  0R-JUMPB  [B0R-JMP]
JP10  JP2W  [JP2W]
JP11  JP1E  [JP1]
JP12  JP2Q  [JP2Q]
JP13  JP1E  [JP1]
JP14  JP1E  [JP1]
R50  10k  R-US_R1206  [R1206]
R51  10k  R-US_R1206  [R1206]
R52  10k  R-US_R1206  [R1206]
R53  10k  R-US_R1206  [R1206]
R54  10k  R-US_R1206  [R1206]
R55  10k  R-US_R1206  [R1206]
R56  10k  R-US_R1206  [R1206]
R57  10k  R-US_R1206  [R1206]
R58  2.2k  R-US_R1206  [R1206]
R59  10M  R-US_R1206  [R1206]
R60  22k  R-US_R1206  [R1206]
R61  22k  R-US_R1206  [R1206]
R62  22k  R-US_R1206  [R1206]
R63  7.5k  R-US_R1206  [R1206]
R64  7.5k  R-US_R1206  [R1206]
R65  47k  R-US_R1206  [R1206]
R66  15k  R-US_R1206  [R1206]
R67  47k  R-US_R1206  [R1206]
R68  15k  R-US_R1206  [R1206]
R69  10k  R-US_R1206  [R1206]
R70  10k  R-US_R1206  [R1206]
R71  10k  R-US_R1206  [R1206]
R72  1k  R-US_R1206  [R1206]
U2  PCF8574AT/3,512  [SOIC127P1032X265-16N]
U3  PCA9548APWR  [SOP65P640X120-24N]
U$9  SSM2126  [DIP48]
U$10  PT2257  [SO08]
U$11  PT2399  [DIL16]
X11  22-23-2031  [22-23-2031]
X14  22-23-2031  [22-23-2031]
X15  22-23-2061  [22-23-2061]

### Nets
3.3V1: C139.1 IC4.2(VOUT) JMP4.1 JMP5.1 JMP6.1 R52.1 U3.24(VCC)
9V: U$10.6(VDD) ; also sheet 1
BYPASS: IC3.9(C) IC3.10(B) U2.12(P7)
CM1: U2.9(P4) U$9.P$20(CM1)
CM2: U2.10(P5) U$9.P$21(CM2)
COUT: C148.2 X15.3
DELAY: IC3.11(A) U2.11(P6)
DELFED: C181.2 IC3.13(X1)
DM1: U2.4(P0) U$9.P$16(DM1)
DM2: U2.5(P1) U$9.P$17(DM2)
DM3: U2.6(P2) U$9.P$18(DM3)
DM4: U2.7(P3) U$9.P$19(DM4)
GND: C139.2 C152.2 C153.2 C154.2 C157.2 C180.2 C182.2 C183.2 C184.2 C185.2 C186.2 C187.+ C188.+ C189.- C190.1 C191.2 IC2.3(A:+IN) IC2.5(B:+IN) IC3.6(INH) IC4.1(GND) JMP4.3 JMP5.3 JMP6.3 JP10.2 R58.2 R59.2 R62.1 R66.2 R68.2 R70.2 U2.8(VSS) U3.12(GND) U$9.P$3(VREF) U$9.P$15(VREF1) U$9.P$22(LREF) U$9.P$38(VREF2) U$10.3(GND) U$11.3(AGND) U$11.4(DGND) X11.2 X14.2 X15.6 ; also sheet 1
LFED: C141.2 U$9.P$9(LIN)
LMIX: IC2.2(A:-IN) R50.1 X14.3 ; also sheet 1
LO1: C146.1 IC3.1(Y1) IC5.5(B:+IN) U$9.P$24(LROT)
LOUT: C146.2 X15.1
LP-: C176.1 C177.2 R71.2 U$11.16(LP1-)
LT: C175.1 U$9.P$8(LT)
N$241: C140.2 IC2.1(A:OUT) R50.2
N$242: C192.1 IC5.1(A:OUT) IC5.2(A:-IN)
N$243: C193.1 IC5.6(B:-IN) IC5.7(B:OUT)
N$244: C142.2 IC2.7(B:OUT) R51.2
N$245: C140.1 U$10.1(LIN)
N$246: C142.1 U$10.8(RIN)
N$247: C141.1 U$10.2(LOUT)
N$248: C143.1 U$10.7(ROUT)
N$249: R52.2 U3.3(~RESET)
N$257: C192.2 X11.1
N$258: JMP5.2 U3.2(A1)
N$260: JMP6.2 U3.21(A2)
N$261: JMP4.2 U3.1(A0)
N$262: IC3.2(Y0) IC3.5(Z0) IC3.14(X)
N$263: R57.2 U2.13(!INT)
N$264: C144.1 IC3.15(Y)
N$265: C145.1 IC3.4(Z)
N$268: C148.1 U$9.P$25(COUT)
N$269: R58.1 U$11.6(VC0)
N$270: C149.1 U$9.P$1(CT5)
N$271: C150.1 U$9.P$2(CT1)
N$272: C151.1 U$9.P$5(CT4)
N$273: C152.1 R59.1 U$9.P$6(CAB)
N$274: R61.2 U$9.P$14(NOUT)
N$278: C153.1 R60.1 U$9.P$11(NIN)
N$279: C193.2 X11.3
N$281: C154.1 C156.2 R60.2 R62.2
N$282: C156.1 R61.1
N$283: C157.1 C187.- U$9.P$23(VRO)
N$284: C158.2 U$9.P$29(CC1)
N$285: C158.1 U$9.P$28(CC2)
N$286: C160.1 U$9.P$31(ACS1)
N$287: C160.2 U$9.P$32(ACS2)
N$289: C159.1 U$9.P$33(ACC1)
N$290: C159.2 U$9.P$34(ACC2)
N$291: C161.1 R63.1 U$9.P$35(ACR1)
N$292: C161.2 U$9.P$36(ACR2)
N$293: C162.2 U$9.P$40(ACL2)
N$294: C162.1 R64.1 U$9.P$39(ACL1)
N$295: C163.2 R65.1 U$9.P$41(BPLIN)
N$296: C166.2 U$9.P$46(CT6)
N$297: C170.2 U$9.P$42(CFWS)
N$298: C169.2 U$9.P$43(CFWC)
N$299: C168.2 U$9.P$44(CFWL)
N$300: C167.2 U$9.P$45(CFWR)
N$301: C165.2 U$9.P$47(CT3)
N$302: C164.2 U$9.P$48(CT2)
N$303: C171.2 R65.2 R66.1
N$304: C171.1 C172.2 R64.2
N$305: C173.2 R67.1 U$9.P$37(BPRIN)
N$306: C174.2 R67.2 R68.1
N$307: C174.1 C175.2 R63.2
N$308: C176.2 R69.2
N$309: C177.1 R71.1 U$11.15(LP1+)
N$310: C178.2 U$11.9(OP1-)
N$311: C179.2 U$11.11(OP2-)
N$312: C178.1 U$11.10(OP1+)
N$313: C179.1 R72.2 U$11.12(OP2+)
N$314: C180.1 C181.1 R72.1
N$315: C183.1 U$11.7(CC1)
N$316: C182.1 U$11.8(CC0)
N$317: C185.1 U$11.2(REF)
N$318: JP13.2 R53.2 U$10.4(SDA)
N$319: JP13.1 R54.1 U$10.5(SCL)
N$320: JP14.2 R56.2 U2.15(SDA)
N$321: JP14.1 R55.2 U2.14(SCL)
RFED: C143.2 U$9.P$10(RIN)
RLOUT: C144.2 X15.4
RMIX: IC2.6(B:-IN) R51.1 X14.1 ; also sheet 1
RO1: C147.1 IC3.3(Z1) IC5.3(A:+IN) U$9.P$26(ROUT)
ROUT: C147.2 X15.2
RROUT: C145.2 X15.5
RT: C172.1 U$9.P$7(RT)
SC0: JP12.1 U3.5(SC0)
SC1: JP12.3 U3.7(SC1)
SCLL: JP11.2 U3.22(SCL)
SD8: JP12.2 U3.4(SD0)
SD9: JP12.4 U3.6(SD1)
SDAA: JP11.1 U3.23(SDA)
SFED: IC3.12(X0) R69.1 R70.1 U$9.P$30(SOUT)
V-: C149.2 C150.2 C151.2 C163.1 C164.1 C165.1 C166.1 C167.1 C168.1 C169.1 C170.1 C173.1 C188.- C190.2 JP10.3 U$9.P$13(V-) U$9.P$27(V--) ; supply symbol labelled VEE
VCC: C184.1 C186.1 C189.+ C191.1 IC4.3(VIN) JP10.1 R53.1 R54.2 R55.1 R56.1 R57.1 U2.1(A0) U2.2(A1) U2.3(A2) U2.16(VDD) U$9.P$4(V+) U$11.1(VCC) ; supply symbol labelled V+ ; also sheet 1
Unconnected: U3.8(SD2) U3.9(SC2) U3.10(SD3) U3.11(SC3) U3.13(SD4) U3.14(SC4) U3.15(SD5) U3.16(SC5) U3.17(SD6) U3.18(SC6) U3.19(SD7) U3.20(SC7) U$9.P$12(NC) U$11.5(CLK) U$11.13(LP2-) U$11.14(LP2+)

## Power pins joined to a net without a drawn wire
GND: IC3.8(GND)
V+: IC2.8(P:V+)
V-: IC2.4(P:V-) IC3.7(VEE) IC5.4(P:V-)
VCC: IC3.16(VCC) IC5.8(P:V+)

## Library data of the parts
C1-C186 C190-C193 = adafruit:C-US: CAPACITOR, American symbol
C187-C189 = adafruit:CPOL-US: POLARIZED CAPACITOR, American symbol
IC1 IC4 = burr-brown:REG1117: 800mA and 1A Low Dropout (LDO) Positive Regulator 1.8V, 2.5V, 2.85V, 3.3V, 5V, and Adj; MPN: REG1117; OC_FARNELL: 1097566; OC_NEWARK: 14P6981
IC2 IC5 = linear:LM358: OP AMP also LM158; LM258; LM2904 Source: http://cache.national.com/ds/LM/LM158.pdf
IC3 = 40xx:4053: Triple 2-channel ANALOG MULTIPLEXER
JMP1-JMP6 = jump-0r-smd:0R-JUMP: SMD 0R 0805 Jumper
JP1 = jumper:JP9Q: JUMPER
JP2-JP9 JP11 JP13 JP14 = jumper:JP1E: JUMPER
JP10 = jumper:JP2W: JUMPER
JP12 = jumper:JP2Q: JUMPER
L1-L8 = inductors:BLM15H: EMIFIL (R) Chip Ferrite Bead for GHz Noise
R1-R72 = adafruit:R-US_: RESISTOR, American symbol
RN1-RN4 = resistor-dil:4R-N: Array Chip Resistor Source: RS Component / Phycomp; OC_FARNELL: unknown; OC_NEWARK: unknown
U1 U3 = PCA9548A:PCA9548APWR: 8-CHANNEL I2C SWITCH WITH RESET; MPN: PCA9548APWR False; OC_FARNELL: 1607855; OC_NEWARK: 22M1602; PACKAGE: TSSOP-24; SUPPLIER: Texas Instruments
U2 = PCF8574A:PCF8574AT/3,512: IC, I/O EXPANDER, 8BIT, 16SOIC; MPN: PCF8574AT/3,512; OC_FARNELL: 2101302; OC_NEWARK: 70R6866; PACKAGE: SOIC-16; SUPPLIER: NXP
U$1-U$8 = adafruit:TDA7439
U$9 = adafruit:SSM2126
U$10 = adafruit:PT2257
U$11 = adafruit:PT2399
X1-X11 X14 = con-molex:22-23-2031: .100" (2.54mm) Center Header - 3 Pin; MF: MOLEX; MPN: 22-23-2031; OC_FARNELL: 1462950; OC_NEWARK: 30C0862
X15 = con-molex:22-23-2061: .100" (2.54mm) Center Header - 6 Pin; MF: MOLEX; MPN: 22-23-2061; OC_FARNELL: 1462922; OC_NEWARK: 27C1933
